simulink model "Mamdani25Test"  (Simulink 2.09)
settings: Solver=ode45  StartTime=0.0  StopTime=10  MaxStep=10  RelTol=1e-3  AbsTol=1e-3
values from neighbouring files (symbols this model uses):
  k_s = 1.1    [Mdata.m]    (also in Mdata25.m)
  T = 2.5    [HdataF.m]    (also in Mdata.m = 0.5; Mdata25.m = 0.5; VdataC.m = 0.25; VdataF.m = 0.25)
  tau = 1    [Mdata.m]    (also in Mdata25.m; VdataC.m = m/kv)
  yd = 1    [Mdata.m]    (also in Mdata25.m)
undefined symbols (not defined in the file or in its folder): sfunyst
libraries: fuzzy x1

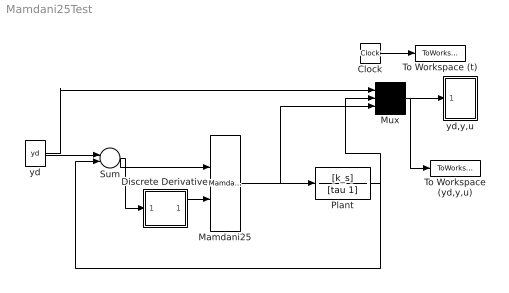
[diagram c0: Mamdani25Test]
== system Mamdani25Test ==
  Clock : Clock
  Discrete Derivative : Subsystem
  Mamdani25 : fuzzy/Mamdani25
  Mux : Mux  Inputs=3
  Plant : TransferFcn  Numerator=[k_s]  Denominator=[tau 1]
  Sum : Sum  Inputs=+-
  To Workspace (yd,y,u) : ToWorkspace  VariableName=yout  SampleTime=0
  To Workspace (t) : ToWorkspace  VariableName=t  SampleTime=0
  yd : Constant  Value=yd
  yd,y,u : Subsystem  mask(Storage scope.){}
      mask help: Storage scope using MATLAB graph window. Enter plotting ranges and line type.
      mask init:
      | npts = @4; color = @5; ax = [0, @1, @2, @3]; dt=-1;
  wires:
  yd/1 -> Mux/1, Sum/1
  Mamdani25/1 -> Plant/1, Mux/3
  Discrete Derivative/1(out_1) -> Mamdani25/2
  Sum/1 -> Discrete Derivative/1(in_1), Mamdani25/1
  Plant/1 -> Mux/2, Sum/2
  Mux/1 -> yd,y,u/1(x), To Workspace (yd,y,u)/1
  Clock/1 -> To Workspace (t)/1

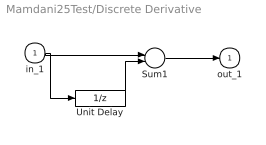
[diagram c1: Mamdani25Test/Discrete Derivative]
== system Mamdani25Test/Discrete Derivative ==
  in_1 : Inport  Port=1  PortWidth=-1  SampleTime=-1
  Sum1 : Sum  Inputs=+-
  Unit Delay : UnitDelay  X0=0  SampleTime=T
  out_1 : Outport  Port=1  InitialOutput=0
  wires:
  Unit Delay/1 -> Sum1/2
  Sum1/1 -> out_1/1
  in_1/1 -> Sum1/1, Unit Delay/1

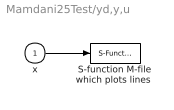
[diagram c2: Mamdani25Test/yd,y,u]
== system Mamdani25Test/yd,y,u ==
  x : Inport  Port=1  PortWidth=-1  SampleTime=-1
  "S-function M-file which plots lines " : S-Function  LoadFcn=sfunyst([],[],[],'LoadBlock')  FunctionName=sfunyst  Parameters=ax, color, npts, dt
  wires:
  x/1 -> "S-function M-file which plots lines "/1
